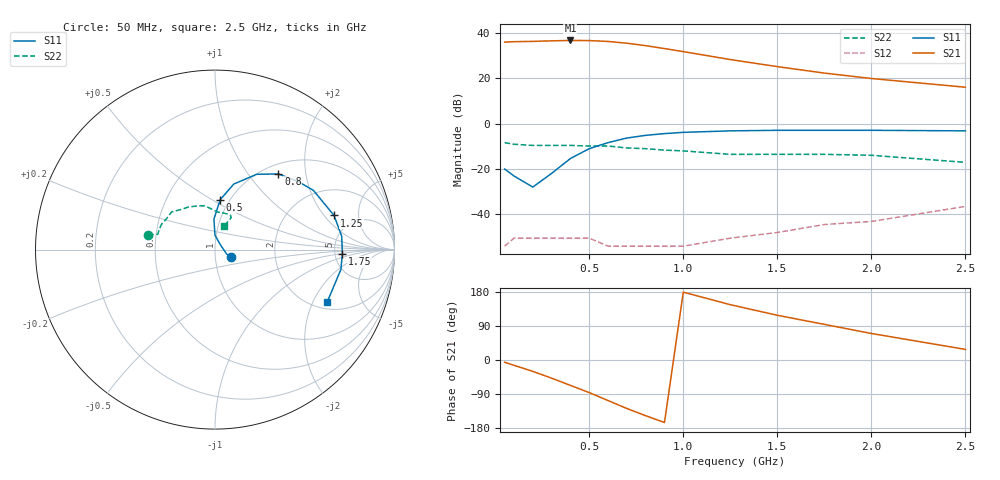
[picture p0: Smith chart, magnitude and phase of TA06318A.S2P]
!  ITA-06318  S PARAMETERS
!  VCC - Vee =5 V  LAST UPDATED 07-22-92
# ghz s ma r 50
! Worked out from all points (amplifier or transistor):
!   16 points, 50 MHz to 2.5 GHz, reference 50 ohm
!   highest |S21| = 36.6 dB at 400 MHz (marker M1)
!   |S21| within 3 dB of that: start of sweep to 855.7 MHz
!   unconditionally stable (mu >= 1): start of sweep to end of sweep
!   at 200 MHz: K = 2.39, MAG = 36.7 dB, |S12| = -50.5 dB
!   at 800 MHz: K = 3.04, MAG = 36.4 dB, |S12| = -54.0 dB
!   at 2.5 GHz: K = 2.86, MAG = 18.8 dB, |S12| = -36.5 dB
!   S11 on the Smith chart (normalised r, x): 50 MHz: 1.20, -0.10; 500 MHz: 0.90, +0.55; 800 MHz: 1.17, +1.42; 1.25 GHz: 3.50, +2.54; 1.75 GHz: 5.84, -0.58; 2.5 GHz: 2.32, -2.59
0.05  0.1 -24.0  62 -6.0  0.002 -104.0  0.38 168.0
0.1  0.07 -21.0  63.3 -14.0  0.003 -86.0  0.35 166.0
0.2  0.04 39.0  64.3 -30.0  0.003 -75.0  0.33 165.0
0.3  0.08 90.0  66.1 -48.0  0.003 -63.0  0.33 161.0
0.4  0.17 92.0  67.4 -67.0  0.003 -57.0  0.33 155.0
0.5  0.28 84.0  67 -86.0  0.003 -44.0  0.32 147.0
0.6  0.38 74.0  64.1 -107.0  0.002 -30.0  0.32 139.0
0.7  0.48 61.0  58.6 -128.0  0.002 -14.0  0.29 129.0
0.8  0.55 50.0  51.8 -147.0  0.002 0.0  0.28 122.0
0.9  0.6 39.0  44.7 -165.0  0.002 16.0  0.26 110.0
1  0.64 31.0  38.3 179.0  0.002 27.0  0.25 103.0
1.25  0.69 16.0  25.6 146.0  0.003 61.0  0.21 86.0
1.5  0.71 6.0  17.9 118.0  0.004 93.0  0.21 73.0
1.75  0.71 -2.0  12.9 94.0  0.006 141.0  0.21 66.0
2  0.71 -9.0  9.8 70.0  0.007 164.0  0.2 63.0
2.5  0.69 -25.0  6.3 28.0  0.015 178.0  0.14 69.0
